| IBIS file imx8qx_17x17_v104.ibs generated by Viper version: 2017.04.12
[IBIS Ver]   6.0
[Comment Char] |_char
[File name]   imx8qxp_17x17_v104.ibs
[File Rev]   1.04
[Date]   Oct 18,2021
[Source]   NXP Viper 2017.04.12
[Notes]
[Disclaimer] IMPORTANT NOTICE
  This information is provided on an AS IS basis and without warranty.
  IN NO EVENT SHALL NXP BE LIABLE FOR INCIDENTAL OR CONSEQUENTIAL
  DAMAGES ARISING FROM USE OF THIS INFORMATION. THIS DISCLAIMER OF
  WARRANTY EXTENDS TO THE USER OF THE INFORMATION, AND TO THEIR CUSTOMERS
  OR USERS OF PRODUCTS  AND IS IN LIEU OF ALL WARRANTIES WHETHER EXPRESS,
  IMPLIED, OR STATUTORY, INCLUDING IMPLIED WARRANTIES OF MERCHANTABILITY
  OR FITNESS FOR PARTICULAR PURPOSE.
  NXP does not represent or warrant that the information furnished
  hereunder is free of infringement of any third party patents,
  copyrights, trade secrets, or other intellectual property rights.
  NXP does not represent or warrant that the information is free of
  defect, or that it meets any particular standard, requirements or need
  of the user of the infomation or their customers.
  NXP reserves the right to change the information in this file
  without notice.
   http://www.nxp.com
[Copyright]   (C) Copyright NXP 2006 - 2018, All Rights Reserved.
|   imx8qxp_17x17
[Component] imx8qxp_17x17_v104
[Manufacturer] NXP
[Package]
|   typ   min   max
R_pkg   0.31846   0.033582   0.75433
L_pkg   2.117e-9   3.409e-10   4.458e-9
C_pkg   1.134e-12   5.597e-13   3.274e-12
[Pin]   Signal_name   model_name   R_pin   L_pin   C_pin
A3   VSS_MAIN   GND   NA   NA   NA
A5   DDR_DCF18   PCKE_PAD   0.60598   3.663e-9   1.638e-12
A7   DDR_CK1_P   PCK_PAD   0.56666   3.47e-9   1.588e-12
A9   DDR_DCF26   PCKE_PAD   0.48689   3.01e-9   1.443e-12
A11   PCIE_CTRL0_PERST_B   3V3SF_1V8_3V3_FCGPIO   0.3033   2.06e-9   1.123e-12
A13   PCIE0_TX0_P   ABI_SERDES   0.34015   2.505e-9   1.009e-12
A15   PCIE0_RX0_P   ABI_SERDES   0.46929   3.272e-9   1.374e-12
A17   USB_OTG1_ID   USB_NXP   0.33178   2.305e-9   1.189e-12
A19   USB_OTG1_DP   USB_NXP   0.36817   2.72e-9   1.1e-12
A21   EMMC0_DATA0   3V3SF_1V8_3V3_FCGPIO   0.40744   2.664e-9   1.313e-12
A23   ENET0_RGMII_RXC   RGMIIRX_GPIO   0.31942   2.189e-9   1.146e-12
A25   ENET0_MDC   3V3SF_1V8_3V3_FCGPIO   0.32796   2.158e-9   1.166e-12
A27   VSS_MAIN   GND   NA   NA   NA
B2   DDR_DCF01   PCKE_PAD   0.68397   4.007e-9   1.734e-12
B4   DDR_DCF07   PCKE_PAD   0.58694   3.527e-9   1.632e-12
B6   DDR_DCF17   PCKE_PAD   0.52931   3.211e-9   1.459e-12
B8   DDR_CK1_N   PCK_PAD   0.59395   3.579e-9   1.611e-12
B10   DDR_DCF21   PCKE_PAD   0.75433   4.458e-9   1.957e-12
B12   PCIE0_TX0_N   ABI_SERDES   0.32805   2.401e-9   1.044e-12
B14   PCIE_CTRL0_WAKE_B   3V3SF_1V8_3V3_FCGPIO   0.37118   2.405e-9   1.258e-12
B16   PCIE0_RX0_N   ABI_SERDES   0.45484   3.105e-9   1.38e-12
B18   USB_OTG1_DN   USB_NXP   0.36895   2.655e-9   1.113e-12
B20   EMMC0_RESET_B   3V3SF_1V8_3V3_FCGPIO   0.3187   2.151e-9   1.117e-12
B22   ENET0_RGMII_TXD3   RGMIITX_GPIO   0.30644   2.133e-9   1.094e-12
B24   ENET0_RGMII_RXD3   RGMIIRX_GPIO   0.30222   2.062e-9   1.102e-12
B26   ESAI0_FSR   RGMIITX_GPIO   0.37989   2.442e-9   1.258e-12
B28   ESAI0_TX4_RX1   RGMIITX_GPIO   0.45602   2.794e-9   1.358e-12
C1   VSS_MAIN   GND   NA   NA   NA
C3   VSS_MAIN   GND   NA   NA   NA
C5   VSS_MAIN   GND   NA   NA   NA
C7   VSS_MAIN   GND   NA   NA   NA
C9   VSS_MAIN   GND   NA   NA   NA
C11   VSS_MAIN   GND   NA   NA   NA
C13   PCIE_REFCLK100M_N   PCIEREFCLKIO_N   0.32064   2.101e-9   1.131e-12
C15   VSS_MAIN   GND   NA   NA   NA
C17   VSS_MAIN   GND   NA   NA   NA
C19   VDD_EMMC0_VSELECT_1P8_3P3   POWER
C21   ENET0_RGMII_TXD1   RGMIITX_GPIO   0.25476   1.777e-9   1.026e-12
C23   ENET0_RGMII_RXD0   RGMIIRX_GPIO   0.28143   1.95e-9   1.063e-12
C25   ESAI0_SCKT   RGMIITX_GPIO   0.32741   2.164e-9   1.13e-12
C27   ESAI0_TX2_RX3   RGMIIRX_GPIO   0.48998   3.038e-9   1.422e-12
C29   VSS_MAIN   GND   NA   NA   NA
D2   DDR_DCF12   PCKE_PAD   0.71074   4.168e-9   1.828e-12
D4   DDR_DCF05   PCKE_PAD   0.5124   3.09e-9   1.489e-12
D6   DDR_DCF20   PCKE_PAD   0.53119   3.213e-9   1.505e-12
D8   DDR_DCF29   PCKE_PAD   0.35048   2.267e-9   1.192e-12
D10   DDR_DCF28   PCKE_PAD   0.4342   2.666e-9   1.32e-12
D12   VDD_USB_3P3   POWER
D14   PCIE_REFCLK100M_P   PCIEREFCLKIO_P   0.32297   2.08e-9   1.168e-12
D16   VDD_USB_SS3_LDO_1P0_CAP   POWER
D18   VDD_EMMC0_1P8_3P3   POWER
D20   VDD_ENET0_VSELECT_1P8_2P5_3P3   POWER
D22   ENET0_RGMII_RXD1   RGMIIRX_GPIO   0.1839   1.421e-9   8.563e-13
D24   ESAI0_TX3_RX2   RGMIIRX_GPIO   0.3864   2.495e-9   1.223e-12
D26   SPI3_CS0   3V3SF_1V8_3V3_FCGPIO   0.54046   3.334e-9   1.559e-12
D28   SPI3_SCK   3V3SF_1V8_3V3_FCGPIO   0.38925   2.486e-9   1.254e-12
E1   DDR_DCF15   PCKE_PAD   0.65321   3.867e-9   1.722e-12
E3   DDR_DCF03   PCKE_PAD   0.50795   3.087e-9   1.474e-12
E5   DDR_DCF22   PCKE_PAD   0.48237   2.951e-9   1.392e-12
E7   DDR_DCF32   PCKE_PAD   0.33907   2.197e-9   1.192e-12
E9   DDR_DCF27   PCKE_PAD   0.32561   2.108e-9   1.154e-12
E11   PCIE_CTRL0_CLKREQ_B   3V3SF_1V8_3V3_FCGPIO   0.16383   1.294e-9   8.23e-13
E13   EMMC0_CMD   3V3SF_1V8_3V3_FCGPIO   0.1937   1.633e-9   9.088e-13
E15   EMMC0_DATA6   3V3SF_1V8_3V3_FCGPIO   0.3561   2.314e-9   1.223e-12
E17   VSS_MAIN   GND   NA   NA   NA
E19   EMMC0_DATA3   3V3SF_1V8_3V3_FCGPIO   0.2151   1.54e-9   8.782e-13
E21   VDD_ENET0_1P8_2P5_3P3   POWER
E23   ESAI0_FST   RGMIITX_GPIO   0.19585   1.448e-9   9.33e-13
E25   ESAI0_TX1   RGMIIRX_GPIO   0.29822   1.981e-9   1.079e-12
E27   SPDIF0_EXT_CLK   RGMIITX_GPIO   0.34327   2.258e-9   1.153e-12
E29   UART1_RX   3V3SF_1V8_3V3_FCGPIO   0.43258   2.758e-9   1.353e-12
F2   VSS_MAIN   GND   NA   NA   NA
F4   VSS_MAIN   GND   NA   NA   NA
F6   VSS_MAIN   GND   NA   NA   NA
F8   VSS_MAIN   GND   NA   NA   NA
F10   DDR_ZQ   NC   0.20708   1.713e-9   1.28e-12
F12   PCIE_REF_QR   NC   0.17551   1.316e-9   9.358e-13
F14   EMMC0_CLK   3V3SF_1V8_3V3_FCGPIO   0.1708   1.429e-9   8.15e-13
F16   EMMC0_DATA5   3V3SF_1V8_3V3_FCGPIO   0.12694   1.075e-9   7.546e-13
F18   EMMC0_DATA1   3V3SF_1V8_3V3_FCGPIO   0.16418   1.28e-9   8.764e-13
F20   ENET0_RGMII_TXD0   RGMIITX_GPIO   0.19161   1.414e-9   8.951e-13
F22   ENET0_REFCLK_125M_25M   3V3SF_1V8_3V3_FCGPIO   0.16413   1.301e-9   7.971e-13
F24   SPDIF0_RX   RGMIIRX_GPIO   0.28282   1.891e-9   1.046e-12
F26   VDD_ENET_MDIO_1P8_3P3   POWER
F28   SPI3_CS1   3V3SF_1V8_3V3_FCGPIO   0.35831   2.326e-9   1.185e-12
G1   DDR_DCF10   PCKE_PAD   0.65109   3.855e-9   1.688e-12
G3   DDR_CK0_N   PCK_PAD   0.55273   3.295e-9   1.525e-12
G5   DDR_DCF00   PCKE_PAD   0.49032   2.993e-9   1.45e-12
G7   DDR_DCF33   PCKE_PAD   0.31582   2.024e-9   1.17e-12
G9   DDR_DCF31   PCKE_PAD   0.3963   2.501e-9   1.183e-12
G11   PCIE0_PHY_PLL_REF_RETURN   GND   0.033582   5.677e-10   1.252e-12
G13   USB_SS3_TC1   3V3SF_3V3_FCGPIO   0.11957   1.018e-9   7.88e-13
G15   EMMC0_DATA2   3V3SF_1V8_3V3_FCGPIO   0.14436   1.152e-9   7.231e-13
G17   EMMC0_DATA4   3V3SF_1V8_3V3_FCGPIO   0.14044   1.144e-9   8.112e-13
G19   ENET0_RGMII_TXC   RGMIITX_GPIO   0.14473   1.165e-9   8.155e-13
G21   ENET0_RGMII_RXD2   RGMIIRX_GPIO   0.14641   1.239e-9   7.478e-13
G23   ESAI0_TX0   RGMIIRX_GPIO   0.21582   1.512e-9   9.211e-13
G25   SPI3_SDO   3V3SF_1V8_3V3_FCGPIO   0.28321   1.89e-9   1.032e-12
G27   UART1_CTS_B   3V3SF_1V8_3V3_FCGPIO   0.34681   2.245e-9   1.16e-12
G29   UART1_RTS_B   3V3SF_1V8_3V3_FCGPIO   0.37578   2.468e-9   1.258e-12
H2   DDR_CK0_P   PCK_PAD   0.51499   3.138e-9   1.476e-12
H4   DDR_DCF24   PCKE_PAD   0.37984   2.355e-9   1.21e-12
H6   DDR_DCF19   PCKE_PAD   0.34619   2.213e-9   1.204e-12
H8   DDR_DCF30   PCKE_PAD   0.24305   1.688e-9   1.007e-12
H10   DDR_DCF25   PCKE_PAD   0.32921   2.167e-9   1.178e-12
H12   PCIE_REXT   NC   0.093831   8.543e-10   6.92e-13
H14   USB_SS3_TC3   3V3SF_3V3_FCGPIO   0.11822   1.017e-9   7.579e-13
H16   EMMC0_DATA7   3V3SF_1V8_3V3_FCGPIO   0.08452   8.213e-10   7.472e-13
H18   ENET0_RGMII_TX_CTL   RGMIITX_GPIO   0.046311   6.292e-10   5.597e-13
H20   ENET0_RGMII_RX_CTL   RGMIIRX_GPIO   0.19545   1.425e-9   8.908e-13
H22   ESAI0_SCKR   RGMIITX_GPIO   0.16182   1.249e-9   7.9e-13
H24   SPI3_SDI   3V3SF_1V8_3V3_FCGPIO   0.29834   1.966e-9   1.068e-12
H26   VSS_MAIN   GND   NA   NA   NA
H28   SPI0_CS0   3V3SF_1V8_3V3_FCGPIO   0.42978   2.766e-9   1.304e-12
J1   VSS_MAIN   GND   NA   NA   NA
J3   VSS_MAIN   GND   NA   NA   NA
J5   VSS_MAIN   GND   NA   NA   NA
J7   VSS_MAIN   GND   NA   NA   NA
J9   VDD_PCIE_DIG_1P8_3P3   POWER
J11   VDD_PCIE_1P8   POWER
J13   VSS_MAIN   GND   NA   NA   NA
J15   USB_OTG1_VBUS   USB_NXP   0.13315   1.223e-9   6.609e-13
J17   EMMC0_STROBE   3V3SF_1V8_3V3_FCGPIO   0.074471   7.722e-10   6.943e-13
J19   ENET0_RGMII_TXD2   RGMIITX_GPIO   0.038799   3.409e-10   6.494e-13
J21   ENET0_MDIO   3V3SF_1V8_3V3_FCGPIO   0.10797   9.439e-10   7.106e-13
J23   SPDIF0_TX   RGMIIRX_GPIO   0.22123   1.614e-9   9.35e-13
J25   UART1_TX   3V3SF_1V8_3V3_FCGPIO   0.30141   1.998e-9   1.09e-12
J27   SPI0_SDO   3V3SF_1V8_3V3_FCGPIO   0.31847   2.065e-9   1.139e-12
J29   SPI0_SDI   3V3SF_1V8_3V3_FCGPIO   0.34645   2.267e-9   1.203e-12
K2   DDR_DCF08   PCKE_PAD   0.47957   2.948e-9   1.473e-12
K4   DDR_DCF14   PCKE_PAD   0.4787   2.939e-9   1.452e-12
K6   DDR_DCF04   PCKE_PAD   0.25956   1.689e-9   9.947e-13
K8   VDD_DDR_VDDQ   POWER
K10   VDD_ANA0_1P8   POWER
K12   VDD_PCIE_LDO_1P0_CAP   POWER
K14   VDD_USB_1P8   POWER
K16   VDD_MAIN   POWER
K18   VSS_MAIN   GND   NA   NA   NA
K20   VDD_GPU   POWER
K22   ESAI0_TX5_RX0   RGMIITX_GPIO   0.18734   1.405e-9   8.834e-13
K24   MCLK_OUT0   3V3SF_1V8_3V3_FCGPIO   0.27272   1.839e-9   1.066e-12
K26   VDD_ESAI_SPDIF_1P8_2P5_3P3   POWER
K28   SPI0_CS1   3V3SF_1V8_3V3_FCGPIO   0.32295   2.115e-9   1.146e-12
L1   DDR_DCF11   PCKE_PAD   0.39285   2.474e-9   1.275e-12
L3   DDR_DCF09   PCKE_PAD   0.43975   2.731e-9   1.384e-12
L5   DDR_DCF23   PCKE_PAD   0.25824   1.745e-9   1.009e-12
L7   DDR_DCF16   PCKE_PAD   0.25409   1.709e-9   9.506e-13
L9   VSS_MAIN   GND   NA   NA   NA
L11   VSS_MAIN   GND   NA   NA   NA
L13   VDD_MAIN   POWER
L15   VSS_MAIN   GND   NA   NA   NA
L17   VDD_GPU   POWER
L19   VDD_GPU   POWER
L21   VDD_MAIN   POWER
L23   MCLK_IN0   3V3SF_1V8_3V3_FCGPIO   0.14369   1.143e-9   7.893e-13
L25   SPI0_SCK   3V3SF_1V8_3V3_FCGPIO   0.19113   1.427e-9   9.442e-13
L27   VDD_SPI_MCLK_UART_1P8_3P3   POWER
L29   VSS_MAIN   GND   NA   NA   NA
M2   VSS_MAIN   GND   NA   NA   NA
M4   VSS_MAIN   GND   NA   NA   NA
M6   VSS_MAIN   GND   NA   NA   NA
M8   VDD_DDR_VDDQ   POWER
M10   VDD_MAIN   POWER
M12   VSS_MAIN   GND   NA   NA   NA
M14   VDD_MAIN   POWER
M16   VSS_MAIN   GND   NA   NA   NA
M18   VDD_GPU   POWER
M20   VSS_MAIN   GND   NA   NA   NA
M22   MCLK_IN1   3V3SF_1V8_3V3_FCGPIO   0.10409   9.11e-10   7.793e-13
M24   VSS_MAIN   GND   NA   NA   NA
M26   VSS_MAIN   GND   NA   NA   NA
M28   ADC_VREFH   POWER   0.19187   1.497e-9   1.547e-12
N1   DDR_DQ02   PDDRIO_PAD   0.55563   3.352e-9   1.521e-12
N3   DDR_DQ00   PDDRIO_PAD   0.50424   3.21e-9   1.442e-12
N5   DDR_DQ13   PDDRIO_PAD   0.45478   2.757e-9   1.37e-12
N7   DDR_DQ15   PDDRIO_PAD   0.35806   2.282e-9   1.073e-12
N9   VDD_DDR_VDDQ   POWER
N11   VDD_MAIN   POWER
N13   VSS_MAIN   GND   NA   NA   NA
N15   VDD_MAIN   POWER
N17   VSS_MAIN   GND   NA   NA   NA
N19   VDD_GPU   POWER
N21   VSS_MAIN   GND   NA   NA   NA
N23   ADC_IN1   CSF_1V8_FCGPIO   0.15303   1.165e-9   8.275e-13
N25   ADC_IN3   CSF_1V8_FCGPIO   0.26276   1.717e-9   9.703e-13
N27   ADC_IN2   CSF_1V8_FCGPIO   0.25756   1.755e-9   9.937e-13
N29   ADC_VREFL   GND   0.17561   1.455e-9   1.639e-12
P2   DDR_DQ01   PDDRIO_PAD   0.40818   2.601e-9   1.24e-12
P4   DDR_DQ12   PDDRIO_PAD   0.31857   2.054e-9   1.081e-12
P6   DDR_DQ14   PDDRIO_PAD   0.32363   2.082e-9   1.079e-12
P8   VDD_DDR_VDDQ   POWER
P10   VSS_MAIN   GND   NA   NA   NA
P12   VDD_MAIN   POWER
P14   VSS_MAIN   GND   NA   NA   NA
P16   VDD_MAIN   POWER
P18   VSS_MAIN   GND   NA   NA   NA
P20   VDD_GPU   POWER
P22   VDD_ADC_1P8   POWER
P24   ADC_IN0   CSF_1V8_FCGPIO   0.17153   1.276e-9   8.767e-13
P26   ADC_IN5   CSF_1V8_FCGPIO   0.23782   1.642e-9   9.683e-13
P28   ADC_IN4   CSF_1V8_FCGPIO   0.27134   1.832e-9   1.061e-12
R1   VSS_MAIN   GND   NA   NA   NA
R3   VSS_MAIN   GND   NA   NA   NA
R5   VSS_MAIN   GND   NA   NA   NA
R7   VSS_MAIN   GND   NA   NA   NA
R9   VSS_MAIN   GND   NA   NA   NA
R11   VSS_MAIN   GND   NA   NA   NA
R13   VDD_MAIN   POWER
R15   VSS_MAIN   GND   NA   NA   NA
R17   VDD_GPU   POWER
R19   VSS_MAIN   GND   NA   NA   NA
R21   VDD_MAIN   POWER
R23   VSS_MAIN   GND   NA   NA   NA
R25   VSS_MAIN   GND   NA   NA   NA
R27   VSS_MAIN   GND   NA   NA   NA
R29   VSS_MAIN   GND   NA   NA   NA
T2   DDR_DQ03   PDDRIO_PAD   0.37672   2.394e-9   1.21e-12
T4   DDR_DQS1_N   PDQS_PAD   0.33781   2.201e-9   1.025e-12
T6   DDR_DM1   PDDRIO_PAD   0.16039   1.193e-9   7.698e-13
T8   VDD_DDR_VDDQ   POWER
T10   VDD_MAIN   POWER
T12   VSS_MAIN   GND   NA   NA   NA
T14   VDD_MAIN   POWER
T16   VSS_MAIN   GND   NA   NA   NA
T18   VDD_GPU   POWER
T20   VSS_MAIN   GND   NA   NA   NA
T22   FLEXCAN0_RX   3V3SF_1V8_3V3_FCGPIO   0.35436   2.283e-9   1.246e-12
T24   FLEXCAN1_RX   3V3SF_1V8_3V3_FCGPIO   0.27694   1.832e-9   1.042e-12
T26   VDD_ADC_DIG_1P8   POWER
T28   FLEXCAN2_RX   3V3SF_1V8_3V3_FCGPIO   0.2951   1.929e-9   1.093e-12
U1   DDR_DQS0_N   PDQS_PAD   0.50661   3.092e-9   1.537e-12
U3   DDR_DQS0_P   PDQS_PAD   0.53219   3.191e-9   1.464e-12
U5   DDR_DQS1_P   PDQS_PAD   0.31801   2.083e-9   1.001e-12
U7   DDR_DTO0   PDDRIO_PAD   0.098895   8.797e-10   7.121e-13
U9   VDD_DDR_VDDQ   POWER
U11   VDD_MAIN   POWER
U13   VSS_MAIN   GND   NA   NA   NA
U15   VDD_MAIN   POWER
U17   VSS_MAIN   GND   NA   NA   NA
U19   VDD_MAIN   POWER
U21   VDD_CAN_UART_1P8_3P3   POWER
U23   UART0_TX   3V3SF_1V8_3V3_FCGPIO   0.19876   1.443e-9   8.795e-13
U25   FLEXCAN0_TX   3V3SF_1V8_3V3_FCGPIO   0.31323   2.004e-9   1.087e-12
U27   FLEXCAN2_TX   3V3SF_1V8_3V3_FCGPIO   0.24294   1.671e-9   8.827e-13
U29   FLEXCAN1_TX   3V3SF_1V8_3V3_FCGPIO   0.27629   1.907e-9   1.1e-12
V2   VSS_MAIN   GND   NA   NA   NA
V4   VSS_MAIN   GND   NA   NA   NA
V6   VSS_MAIN   GND   NA   NA   NA
V8   VDD_DDR_VDDQ   POWER
V10   VSS_MAIN   GND   NA   NA   NA
V12   VDD_A35   POWER
V14   VDD_A35   POWER
V16   VDD_A35   POWER
V18   VSS_MAIN   GND   NA   NA   NA
V20   VDD_MAIN   POWER
V22   MIPI_DSI0_I2C0_SDA   3V3SF_1V8_3V3_FCGPIO   0.076086   7.914e-10   6.572e-13
V24   VSS_MAIN   GND   NA   NA   NA
V26   UART2_TX   3V3SF_1V8_3V3_FCGPIO   0.17121   1.271e-9   8.781e-13
V28   UART0_RX   3V3SF_1V8_3V3_FCGPIO   0.26081   1.794e-9   9.544e-13
W1   DDR_DM0   PDDRIO_PAD   0.35899   2.276e-9   1.198e-12
W3   DDR_DQ10   PDDRIO_PAD   0.23291   1.571e-9   8.963e-13
W5   DDR_ATO   NC   0.37202   2.325e-9   1.123e-12
W7   VDD_DDR_PLL_1P8   POWER
W9   VSS_MAIN   GND   NA   NA   NA
W11   VSS_MAIN   GND   NA   NA   NA
W13   VDD_A35   POWER
W15   VDD_A35   POWER
W17   VDD_A35   POWER
W19   VSS_MAIN   GND   NA   NA   NA
W21   VDD_ANA1_1P8   POWER
W23   JTAG_TMS   CSF_1V8_FCGPIO   0.17649   1.322e-9   8.415e-13
W25   MIPI_DSI1_I2C0_SDA   3V3SF_1V8_3V3_FCGPIO   0.18746   1.357e-9   8.589e-13
W27   MIPI_DSI0_I2C0_SCL   3V3SF_1V8_3V3_FCGPIO   0.21768   1.557e-9   9.53e-13
W29   UART2_RX   3V3SF_1V8_3V3_FCGPIO   0.30148   2.093e-9   1.126e-12
Y2   DDR_DQ04   PDDRIO_PAD   0.33834   2.165e-9   1.187e-12
Y4   DDR_DQ08   PDDRIO_PAD   0.18397   1.396e-9   8.449e-13
Y6   DDR_VREF   POWER   0.047878   4.824e-10   3.274e-12
Y8   VDD_DDR_VDDQ   POWER
Y10   VDD_MAIN   POWER
Y12   VSS_MAIN   GND   NA   NA   NA
Y14   VDD_MAIN   POWER
Y16   VSS_MAIN   GND   NA   NA   NA
Y18   VDD_MAIN   POWER
Y20   VSS_MAIN   GND   NA   NA   NA
Y22   SCU_GPIO0_00   CSF_1V8_FCGPIO   0.14821   1.137e-9   8.116e-13
Y24   JTAG_TDO   CSF_1V8_FCGPIO   0.27697   1.856e-9   1.043e-12
Y26   VDD_SNVS_4P2   POWER
Y28   MIPI_DSI1_I2C0_SCL   3V3SF_1V8_3V3_FCGPIO   0.27823   1.915e-9   1.042e-12
AA1   VSS_MAIN   GND   NA   NA   NA
AA3   VSS_MAIN   GND   NA   NA   NA
AA5   VSS_MAIN   GND   NA   NA   NA
AA7   VSS_MAIN   GND   NA   NA   NA
AA9   VDD_DDR_VDDQ   POWER
AA11   VDD_MAIN   POWER
AA13   VDD_MIPI_1P8   POWER
AA15   VDD_MIPI_1P0   POWER
AA17   VSS_MAIN   GND   NA   NA   NA
AA19   VDD_MAIN   POWER
AA21   VDD_TMPR_CSI_1P8_3P3   POWER
AA23   PMIC_INT_B   CSF_1V8_FCGPIO   0.23793   1.675e-9   9.771e-13
AA25   TEST_MODE_SELECT   CSF_1V8_FCGPIO   0.25321   1.727e-9   9.528e-13
AA27   VSS_MAIN   GND   NA   NA   NA
AA29   JTAG_TCK   CSF_1V8_FCGPIO   0.32393   2.149e-9   1.169e-12
AB2   DDR_DQ05   PDDRIO_PAD   0.31478   1.975e-9   1.073e-12
AB4   DDR_DQ11   PDDRIO_PAD   0.31536   2.062e-9   1.079e-12
AB6   DDR_DTO1   PDDRIO_PAD   0.30358   1.978e-9   1.084e-12
AB8   VDD_DDR_VDDQ   POWER
AB10   QSPI0A_DQS   3V3SF_1V8_3V3_FCGPIO   0.16544   1.252e-9   7.974e-13
AB12   QSPI0A_SS0_B   3V3SF_1V8_3V3_FCGPIO   0.12301   1.068e-9   7.379e-13
AB14   VDD_MIPI_1P8   POWER
AB16   VDD_MIPI_1P0   POWER
AB18   VDD_MIPI_CSI_DIG_1P8   POWER
AB20   PMIC_ON_REQ   IO_20UM_RES_ANAF_1V8   0.25377   1.732e-9   1.015e-12
AB22   SCU_BOOT_MODE3   CSF_1V8_FCGPIO   0.14142   1.539e-9   7.172e-13
AB24   SCU_PMIC_STANDBY   CSF_1V8_FCGPIO   0.39697   2.526e-9   1.282e-12
AB26   VDD_SNVS_LDO_1P8_CAP   POWER
AB28   JTAG_TRST_B   CSF_1V8_FCGPIO   0.2837   1.928e-9   1.052e-12
AC1   DDR_DQ06   PDDRIO_PAD   0.34319   2.15e-9   1.174e-12
AC3   DDR_DQ07   PDDRIO_PAD   0.30034   1.943e-9   9.997e-13
AC5   DDR_DQ09   PDDRIO_PAD   0.27828   1.992e-9   9.843e-13
AC7   QSPI0B_DATA0   3V3SF_1V8_3V3_FCGPIO   0.20931   1.491e-9   9.385e-13
AC9   QSPI0A_DATA2   3V3SF_1V8_3V3_FCGPIO   0.19074   1.515e-9   8.42e-13
AC11   MIPI_CSI0_DATA3_N   MIPI_CSI   0.36497   2.357e-9   1.219e-12
AC13   MIPI_CSI0_DATA1_N   MIPI_CSI   0.37028   2.387e-9   1.176e-12
AC15   MIPI_CSI0_CLK_N   MIPI_CSI   0.33094   2.141e-9   1.162e-12
AC17   MIPI_CSI0_DATA0_N   MIPI_CSI   0.3426   2.262e-9   1.078e-12
AC19   MIPI_CSI0_DATA2_N   MIPI_CSI   0.34464   2.341e-9   1.202e-12
AC21   CSI_D00   IO_20UM_RES_ANAF   0.2875   1.926e-9   1.045e-12
AC23   SCU_BOOT_MODE1   CSF_1V8_FCGPIO   0.46828   3.067e-9   1.28e-12
AC25   SCU_GPIO0_01   CSF_1V8_FCGPIO   0.28162   1.859e-9   9.376e-13
AC27   PMIC_I2C_SCL   CSF_1V8_FCGPIO   0.29178   1.969e-9   9.85e-13
AC29   JTAG_TDI   CSF_1V8_FCGPIO   0.36581   2.383e-9   1.201e-12
AD2   VSS_MAIN   GND   NA   NA   NA
AD4   VSS_MAIN   GND   NA   NA   NA
AD6   VSS_MAIN   GND   NA   NA   NA
AD8   VDD_QSPI0A_1P8_3P3   POWER
AD10   QSPI0A_SS1_B   3V3SF_1V8_3V3_FCGPIO   0.21596   1.516e-9   9.282e-13
AD12   MIPI_CSI0_DATA3_P   MIPI_CSI   0.36604   2.336e-9   1.269e-12
AD14   MIPI_CSI0_DATA1_P   MIPI_CSI   0.35133   2.266e-9   1.16e-12
AD16   MIPI_CSI0_CLK_P   MIPI_CSI   0.31792   2.092e-9   1.089e-12
AD18   MIPI_CSI0_DATA0_P   MIPI_CSI   0.33148   2.205e-9   1.186e-12
AD20   MIPI_CSI0_DATA2_P   MIPI_CSI   0.35486   2.319e-9   1.155e-12
AD22   CSI_D02   IO_20UM_RES_ANAF   0.18011   1.338e-9   8.479e-13
AD24   VSS_MAIN   GND   NA   NA   NA
AD26   SCU_BOOT_MODE0   CSF_1V8_FCGPIO   0.26532   1.766e-9   1.036e-12
AD28   POR_B   CSF_1V8_FCGPIO   0.33136   2.163e-9   1.143e-12
AE1   QSPI0B_DATA1   3V3SF_1V8_3V3_FCGPIO   0.43816   2.72e-9   1.339e-12
AE3   QSPI0B_DATA3   3V3SF_1V8_3V3_FCGPIO   0.34172   2.199e-9   1.163e-12
AE5   VDD_QSPI0B_1P8_3P3   POWER
AE7   QSPI0B_SS0_B   3V3SF_1V8_3V3_FCGPIO   0.24295   1.662e-9   9.832e-13
AE9   VSS_MAIN   GND   NA   NA   NA
AE11   VSS_MAIN   GND   NA   NA   NA
AE13   VSS_MAIN   GND   NA   NA   NA
AE15   VSS_MAIN   GND   NA   NA   NA
AE17   VSS_MAIN   GND   NA   NA   NA
AE19   VSS_MAIN   GND   NA   NA   NA
AE21   VSS_MAIN   GND   NA   NA   NA
AE23   ANA_TEST_OUT_P   NC   0.24109   1.768e-9   8.791e-13
AE25   SCU_BOOT_MODE2   CSF_1V8_FCGPIO   0.41153   2.694e-9   1.288e-12
AE27   VSS_MAIN   GND   NA   NA   NA
AE29   PMIC_I2C_SDA   CSF_1V8_FCGPIO   0.42834   2.703e-9   1.339e-12
AF2   QSPI0B_DATA2   3V3SF_1V8_3V3_FCGPIO   0.37719   2.419e-9   1.237e-12
AF4   QSPI0B_DQS   3V3SF_1V8_3V3_FCGPIO   0.30699   2.036e-9   1.154e-12
AF6   QSPI0B_SS1_B   3V3SF_1V8_3V3_FCGPIO   0.36204   2.294e-9   1.201e-12
AF8   MIPI_DSI1_DATA0_N   MIPI_LVDS_DSI   0.37839   2.428e-9   1.277e-12
AF10   MIPI_DSI1_DATA1_N   MIPI_LVDS_DSI   0.36272   2.34e-9   1.211e-12
AF12   MIPI_DSI0_DATA3_N   MIPI_LVDS_DSI   0.3616   2.356e-9   1.209e-12
AF14   MIPI_DSI0_CLK_N   MIPI_LVDS_DSI   0.3301   2.168e-9   1.148e-12
AF16   MIPI_DSI0_DATA2_N   MIPI_LVDS_DSI   0.33145   2.163e-9   1.152e-12
AF18   MIPI_CSI0_MCLK_OUT   CSF_1V8_FCGPIO   0.30216   1.966e-9   1.115e-12
AF20   CSI_VSYNC   IO_20UM_RES_ANAF   0.25355   1.811e-9   9.414e-13
AF22   VDD_CSI_1P8_3P3   POWER
AF24   ANA_TEST_OUT_N   NC   0.25249   1.72e-9   9.774e-13
AF26   RTC_XTALO   IO_20UM_RES_ANAF_1V8   0.2789   1.885e-9   1.06e-12
AF28   XTALO   IO_20UM_RES_ANAF_1V8   0.39297   2.475e-9   1.274e-12
AG1   VSS_MAIN   GND   NA   NA   NA
AG3   QSPI0A_SCLK   3V3SF_1V8_3V3_FCGPIO   0.48374   2.971e-9   1.409e-12
AG5   QSPI0A_DATA3   3V3SF_1V8_3V3_FCGPIO   0.35396   2.317e-9   1.193e-12
AG7   MIPI_DSI1_DATA2_N   MIPI_LVDS_DSI   0.42191   2.679e-9   1.329e-12
AG9   MIPI_DSI1_CLK_N   MIPI_LVDS_DSI   0.39245   2.544e-9   1.298e-12
AG11   MIPI_DSI1_DATA3_N   MIPI_LVDS_DSI   0.36671   2.41e-9   1.194e-12
AG13   MIPI_DSI0_DATA1_N   MIPI_LVDS_DSI   0.34731   2.34e-9   1.17e-12
AG15   MIPI_DSI0_DATA0_N   MIPI_LVDS_DSI   0.33429   2.207e-9   1.146e-12
AG17   VSS_MAIN   GND   NA   NA   NA
AG19   CSI_PCLK   3V3SF_1V8_3V3_FCGPIO   0.28612   2.024e-9   1.02e-12
AG21   CSI_D04   IO_20UM_RES_ANAF   0.24994   1.78e-9   1.018e-12
AG23   CSI_D03   IO_20UM_RES_ANAF   0.25608   1.84e-9   9.907e-13
AG25   VSS_MAIN   GND   NA   NA   NA
AG27   VSS_MAIN   GND   NA   NA   NA
AG29   VSS_MAIN   GND   NA   NA   NA
AH2   QSPI0B_SCLK   3V3SF_1V8_3V3_FCGPIO   0.48208   2.96e-9   1.432e-12
AH4   QSPI0A_DATA1   3V3SF_1V8_3V3_FCGPIO   0.44092   2.815e-9   1.339e-12
AH6   VSS_MAIN   GND   NA   NA   NA
AH8   MIPI_DSI1_DATA0_P   MIPI_LVDS_DSI   0.38646   2.565e-9   1.234e-12
AH10   MIPI_DSI1_DATA1_P   MIPI_LVDS_DSI   0.3636   2.493e-9   1.219e-12
AH12   MIPI_DSI0_DATA3_P   MIPI_LVDS_DSI   0.35841   2.451e-9   1.16e-12
AH14   MIPI_DSI0_CLK_P   MIPI_LVDS_DSI   0.32989   2.222e-9   1.147e-12
AH16   MIPI_DSI0_DATA2_P   MIPI_LVDS_DSI   0.33366   2.227e-9   1.158e-12
AH18   CSI_RESET   3V3SF_1V8_3V3_FCGPIO   0.32447   2.187e-9   1.155e-12
AH20   CSI_HSYNC   IO_20UM_RES_ANAF   0.27429   1.939e-9   1.036e-12
AH22   CSI_D07   IO_20UM_RES_ANAF   0.28957   2.007e-9   1.077e-12
AH24   CSI_D01   IO_20UM_RES_ANAF   0.31604   2.206e-9   1.07e-12
AH26   RTC_XTALI   IO_20UM_RES_ANAF_1V8   0.34993   2.421e-9   1.131e-12
AH28   XTALI   IO_20UM_RES_ANAF_1V8   0.4205   2.629e-9   1.289e-12
AJ3   VSS_MAIN   GND   NA   NA   NA
AJ5   QSPI0A_DATA0   3V3SF_1V8_3V3_FCGPIO   0.41463   2.622e-9   1.323e-12
AJ7   MIPI_DSI1_DATA2_P   MIPI_LVDS_DSI   0.42097   2.693e-9   1.334e-12
AJ9   MIPI_DSI1_CLK_P   MIPI_LVDS_DSI   0.39887   2.692e-9   1.296e-12
AJ11   MIPI_DSI1_DATA3_P   MIPI_LVDS_DSI   0.36426   2.501e-9   1.239e-12
AJ13   MIPI_DSI0_DATA1_P   MIPI_LVDS_DSI   0.34325   2.375e-9   1.196e-12
AJ15   MIPI_DSI0_DATA0_P   MIPI_LVDS_DSI   0.32319   2.224e-9   1.165e-12
AJ17   CSI_EN   3V3SF_1V8_3V3_FCGPIO   0.40826   2.716e-9   1.29e-12
AJ19   CSI_MCLK   3V3SF_1V8_3V3_FCGPIO   0.33181   2.241e-9   1.197e-12
AJ21   CSI_D06   IO_20UM_RES_ANAF   0.30705   2.16e-9   1.092e-12
AJ23   CSI_D05   IO_20UM_RES_ANAF   0.35335   2.423e-9   1.173e-12
AJ25   ON_OFF_BUTTON   IO_20UM_RES_ANAF_1V8   0.37037   2.428e-9   1.197e-12
AJ27   VSS_MAIN   GND   NA   NA   NA
[Pin Mapping]   pulldown_ref   pullup_ref   gnd_clamp_ref   power_clamp_ref
A3   GND   NC   NC   NC
A5   GND   VDD_DDR_VDDQ   GND   VDD_DDR_VDDQ
A7   GND   VDD_DDR_VDDQ   GND   VDD_DDR_VDDQ
A9   GND   VDD_DDR_VDDQ   GND   VDD_DDR_VDDQ
A11   GND   VDD_PCIE_DIG_1P   GND   VDD_PCIE_DIG_1P
A13   GND   VDD_PCIE_LDO_1P   GND   VDD_PCIE_LDO_1P
A15   GND   VDD_PCIE_LDO_1P   GND   VDD_PCIE_LDO_1P
A17   GND   VDD_USB_1P8   GND   VDD_USB_1P8
A19   GND   VDD_USB_1P8   GND   VDD_USB_1P8
A21   GND   VDD_EMMC0_1P8_3   GND   VDD_EMMC0_1P8_3
A23   GND   VDD_ENET0_1P8_2   GND   VDD_ENET0_1P8_2
A25   GND   VDD_ENET_MDIO_1   GND   VDD_ENET_MDIO_1
A27   GND   NC   NC   NC
B2   GND   VDD_DDR_VDDQ   GND   VDD_DDR_VDDQ
B4   GND   VDD_DDR_VDDQ   GND   VDD_DDR_VDDQ
B6   GND   VDD_DDR_VDDQ   GND   VDD_DDR_VDDQ
B8   GND   VDD_DDR_VDDQ   GND   VDD_DDR_VDDQ
B10   GND   VDD_DDR_VDDQ   GND   VDD_DDR_VDDQ
B12   GND   VDD_PCIE_LDO_1P   GND   VDD_PCIE_LDO_1P
B14   GND   VDD_PCIE_DIG_1P   GND   VDD_PCIE_DIG_1P
B16   GND   VDD_PCIE_LDO_1P   GND   VDD_PCIE_LDO_1P
B18   GND   VDD_USB_1P8   GND   VDD_USB_1P8
B20   GND   VDD_EMMC0_VSELE   GND   VDD_EMMC0_VSELE
B22   GND   VDD_ENET0_VSELE   GND   VDD_ENET0_VSELE
B24   GND   VDD_ENET0_1P8_2   GND   VDD_ENET0_1P8_2
B26   GND   VDD_ESAI_SPDIF_   GND   VDD_ESAI_SPDIF_
B28   GND   VDD_ESAI_SPDIF_   GND   VDD_ESAI_SPDIF_
C1   GND   NC   NC   NC
C3   GND   NC   NC   NC
C5   GND   NC   NC   NC
C7   GND   NC   NC   NC
C9   GND   NC   NC   NC
C11   GND   NC   NC   NC
C13   GND   VDD_PCIE_1P8   GND   VDD_PCIE_1P8
C15   GND   NC   NC   NC
C17   GND   NC   NC   NC
C19   NC   VDD_EMMC0_VSELE   NC   NC
C21   GND   VDD_ENET0_VSELE   GND   VDD_ENET0_VSELE
C23   GND   VDD_ENET0_1P8_2   GND   VDD_ENET0_1P8_2
C25   GND   VDD_ESAI_SPDIF_   GND   VDD_ESAI_SPDIF_
C27   GND   VDD_ESAI_SPDIF_   GND   VDD_ESAI_SPDIF_
C29   GND   NC   NC   NC
D2   GND   VDD_DDR_VDDQ   GND   VDD_DDR_VDDQ
D4   GND   VDD_DDR_VDDQ   GND   VDD_DDR_VDDQ
D6   GND   VDD_DDR_VDDQ   GND   VDD_DDR_VDDQ
D8   GND   VDD_DDR_VDDQ   GND   VDD_DDR_VDDQ
D10   GND   VDD_DDR_VDDQ   GND   VDD_DDR_VDDQ
D12   NC   VDD_USB_3P3   NC   NC
D14   GND   VDD_PCIE_1P8   GND   VDD_PCIE_1P8
D16   NC   VDD_USB_SS3_LDO   NC   NC
D18   NC   VDD_EMMC0_1P8_3   NC   NC
D20   NC   VDD_ENET0_VSELE   NC   NC
D22   GND   VDD_ENET0_1P8_2   GND   VDD_ENET0_1P8_2
D24   GND   VDD_ESAI_SPDIF_   GND   VDD_ESAI_SPDIF_
D26   GND   VDD_SPI_MCLK_UA   GND   VDD_SPI_MCLK_UA
D28   GND   VDD_SPI_MCLK_UA   GND   VDD_SPI_MCLK_UA
E1   GND   VDD_DDR_VDDQ   GND   VDD_DDR_VDDQ
E3   GND   VDD_DDR_VDDQ   GND   VDD_DDR_VDDQ
E5   GND   VDD_DDR_VDDQ   GND   VDD_DDR_VDDQ
E7   GND   VDD_DDR_VDDQ   GND   VDD_DDR_VDDQ
E9   GND   VDD_DDR_VDDQ   GND   VDD_DDR_VDDQ
E11   GND   VDD_PCIE_DIG_1P   GND   VDD_PCIE_DIG_1P
E13   GND   VDD_EMMC0_1P8_3   GND   VDD_EMMC0_1P8_3
E15   GND   VDD_EMMC0_VSELE   GND   VDD_EMMC0_VSELE
E17   GND   NC   NC   NC
E19   GND   VDD_EMMC0_1P8_3   GND   VDD_EMMC0_1P8_3
E21   NC   VDD_ENET0_1P8_2   NC   NC
E23   GND   VDD_ESAI_SPDIF_   GND   VDD_ESAI_SPDIF_
E25   GND   VDD_ESAI_SPDIF_   GND   VDD_ESAI_SPDIF_
E27   GND   VDD_ESAI_SPDIF_   GND   VDD_ESAI_SPDIF_
E29   GND   VDD_SPI_MCLK_UA   GND   VDD_SPI_MCLK_UA
F2   GND   NC   NC   NC
F4   GND   NC   NC   NC
F6   GND   NC   NC   NC
F8   GND   NC   NC   NC
F10   NC   NC   NC   NC
F12   NC   NC   NC   NC
F14   GND   VDD_EMMC0_1P8_3   GND   VDD_EMMC0_1P8_3
F16   GND   VDD_EMMC0_VSELE   GND   VDD_EMMC0_VSELE
F18   GND   VDD_EMMC0_1P8_3   GND   VDD_EMMC0_1P8_3
F20   GND   VDD_ENET0_VSELE   GND   VDD_ENET0_VSELE
F22   GND   VDD_ENET_MDIO_1   GND   VDD_ENET_MDIO_1
F24   GND   VDD_ESAI_SPDIF_   GND   VDD_ESAI_SPDIF_
F26   NC   VDD_ENET_MDIO_1   NC   NC
F28   GND   VDD_SPI_MCLK_UA   GND   VDD_SPI_MCLK_UA
G1   GND   VDD_DDR_VDDQ   GND   VDD_DDR_VDDQ
G3   GND   VDD_DDR_VDDQ   GND   VDD_DDR_VDDQ
G5   GND   VDD_DDR_VDDQ   GND   VDD_DDR_VDDQ
G7   GND   VDD_DDR_VDDQ   GND   VDD_DDR_VDDQ
G9   GND   VDD_DDR_VDDQ   GND   VDD_DDR_VDDQ
G11   PCIE0_PHY_PLL_R NC   NC   NC
G13   GND   VDD_USB_3P3   GND   VDD_USB_3P3
G15   GND   VDD_EMMC0_1P8_3   GND   VDD_EMMC0_1P8_3
G17   GND   VDD_EMMC0_VSELE   GND   VDD_EMMC0_VSELE
G19   GND   VDD_ENET0_VSELE   GND   VDD_ENET0_VSELE
G21   GND   VDD_ENET0_1P8_2   GND   VDD_ENET0_1P8_2
G23   GND   VDD_ESAI_SPDIF_   GND   VDD_ESAI_SPDIF_
G25   GND   VDD_SPI_MCLK_UA   GND   VDD_SPI_MCLK_UA
G27   GND   VDD_SPI_MCLK_UA   GND   VDD_SPI_MCLK_UA
G29   GND   VDD_SPI_MCLK_UA   GND   VDD_SPI_MCLK_UA
H2   GND   VDD_DDR_VDDQ   GND   VDD_DDR_VDDQ
H4   GND   VDD_DDR_VDDQ   GND   VDD_DDR_VDDQ
H6   GND   VDD_DDR_VDDQ   GND   VDD_DDR_VDDQ
H8   GND   VDD_DDR_VDDQ   GND   VDD_DDR_VDDQ
H10   GND   VDD_DDR_VDDQ   GND   VDD_DDR_VDDQ
H12   NC   NC   NC   NC
H14   GND   VDD_USB_3P3   GND   VDD_USB_3P3
H16   GND   VDD_EMMC0_VSELE   GND   VDD_EMMC0_VSELE
H18   GND   VDD_ENET0_VSELE   GND   VDD_ENET0_VSELE
H20   GND   VDD_ENET0_1P8_2   GND   VDD_ENET0_1P8_2
H22   GND   VDD_ESAI_SPDIF_   GND   VDD_ESAI_SPDIF_
H24   GND   VDD_SPI_MCLK_UA   GND   VDD_SPI_MCLK_UA
H26   GND   NC   NC   NC
H28   GND   VDD_SPI_MCLK_UA   GND   VDD_SPI_MCLK_UA
J1   GND   NC   NC   NC
J3   GND   NC   NC   NC
J5   GND   NC   NC   NC
J7   GND   NC   NC   NC
J9   NC   VDD_PCIE_DIG_1P   NC   NC
J11   NC   VDD_PCIE_1P8   NC   NC
J13   GND   NC   NC   NC
J15   GND   VDD_USB_1P8   GND   VDD_USB_1P8
J17   GND   VDD_EMMC0_VSELE   GND   VDD_EMMC0_VSELE
J19   GND   VDD_ENET0_VSELE   GND   VDD_ENET0_VSELE
J21   GND   VDD_ENET_MDIO_1   GND   VDD_ENET_MDIO_1
J23   GND   VDD_ESAI_SPDIF_   GND   VDD_ESAI_SPDIF_
J25   GND   VDD_SPI_MCLK_UA   GND   VDD_SPI_MCLK_UA
J27   GND   VDD_SPI_MCLK_UA   GND   VDD_SPI_MCLK_UA
J29   GND   VDD_SPI_MCLK_UA   GND   VDD_SPI_MCLK_UA
K2   GND   VDD_DDR_VDDQ   GND   VDD_DDR_VDDQ
K4   GND   VDD_DDR_VDDQ   GND   VDD_DDR_VDDQ
K6   GND   VDD_DDR_VDDQ   GND   VDD_DDR_VDDQ
K8   NC   VDD_DDR_VDDQ   NC   NC
K10   NC   VDD_ANA0_1P8   NC   NC
K12   NC   VDD_PCIE_LDO_1P   NC   NC
K14   NC   VDD_USB_1P8   NC   NC
K16   NC   VDD_MAIN   NC   NC
K18   GND   NC   NC   NC
K20   NC   VDD_GPU   NC   NC
K22   GND   VDD_ESAI_SPDIF_   GND   VDD_ESAI_SPDIF_
K24   GND   VDD_SPI_MCLK_UA   GND   VDD_SPI_MCLK_UA
K26   NC   VDD_ESAI_SPDIF_   NC   NC
K28   GND   VDD_SPI_MCLK_UA   GND   VDD_SPI_MCLK_UA
L1   GND   VDD_DDR_VDDQ   GND   VDD_DDR_VDDQ
L3   GND   VDD_DDR_VDDQ   GND   VDD_DDR_VDDQ
L5   GND   VDD_DDR_VDDQ   GND   VDD_DDR_VDDQ
L7   GND   VDD_DDR_VDDQ   GND   VDD_DDR_VDDQ
L9   GND   NC   NC   NC
L11   GND   NC   NC   NC
L13   NC   VDD_MAIN   NC   NC
L15   GND   NC   NC   NC
L17   NC   VDD_GPU   NC   NC
L19   NC   VDD_GPU   NC   NC
L21   NC   VDD_MAIN   NC   NC
L23   GND   VDD_SPI_MCLK_UA   GND   VDD_SPI_MCLK_UA
L25   GND   VDD_SPI_MCLK_UA   GND   VDD_SPI_MCLK_UA
L27   NC   VDD_SPI_MCLK_UA   NC   NC
L29   GND   NC   NC   NC
M2   GND   NC   NC   NC
M4   GND   NC   NC   NC
M6   GND   NC   NC   NC
M8   NC   VDD_DDR_VDDQ   NC   NC
M10   NC   VDD_MAIN   NC   NC
M12   GND   NC   NC   NC
M14   NC   VDD_MAIN   NC   NC
M16   GND   NC   NC   NC
M18   NC   VDD_GPU   NC   NC
M20   GND   NC   NC   NC
M22   GND   VDD_SPI_MCLK_UA   GND   VDD_SPI_MCLK_UA
M24   GND   NC   NC   NC
M26   GND   NC   NC   NC
M28   NC   ADC_VREFH   NC   NC
N1   GND   VDD_DDR_VDDQ   GND   VDD_DDR_VDDQ
N3   GND   VDD_DDR_VDDQ   GND   VDD_DDR_VDDQ
N5   GND   VDD_DDR_VDDQ   GND   VDD_DDR_VDDQ
N7   GND   VDD_DDR_VDDQ   GND   VDD_DDR_VDDQ
N9   NC   VDD_DDR_VDDQ   NC   NC
N11   NC   VDD_MAIN   NC   NC
N13   GND   NC   NC   NC
N15   NC   VDD_MAIN   NC   NC
N17   GND   NC   NC   NC
N19   NC   VDD_GPU   NC   NC
N21   GND   NC   NC   NC
N23   GND   VDD_ADC_DIG_1P8   GND   VDD_ADC_DIG_1P8
N25   GND   VDD_ADC_DIG_1P8   GND   VDD_ADC_DIG_1P8
N27   GND   VDD_ADC_DIG_1P8   GND   VDD_ADC_DIG_1P8
N29   ADC_VREFL   NC   NC   NC
P2   GND   VDD_DDR_VDDQ   GND   VDD_DDR_VDDQ
P4   GND   VDD_DDR_VDDQ   GND   VDD_DDR_VDDQ
P6   GND   VDD_DDR_VDDQ   GND   VDD_DDR_VDDQ
P8   NC   VDD_DDR_VDDQ   NC   NC
P10   GND   NC   NC   NC
P12   NC   VDD_MAIN   NC   NC
P14   GND   NC   NC   NC
P16   NC   VDD_MAIN   NC   NC
P18   GND   NC   NC   NC
P20   NC   VDD_GPU   NC   NC
P22   NC   VDD_ADC_1P8   NC   NC
P24   GND   VDD_ADC_DIG_1P8   GND   VDD_ADC_DIG_1P8
P26   GND   VDD_ADC_DIG_1P8   GND   VDD_ADC_DIG_1P8
P28   GND   VDD_ADC_DIG_1P8   GND   VDD_ADC_DIG_1P8
R1   GND   NC   NC   NC
R3   GND   NC   NC   NC
R5   GND   NC   NC   NC
R7   GND   NC   NC   NC
R9   GND   NC   NC   NC
R11   GND   NC   NC   NC
R13   NC   VDD_MAIN   NC   NC
R15   GND   NC   NC   NC
R17   NC   VDD_GPU   NC   NC
R19   GND   NC   NC   NC
R21   NC   VDD_MAIN   NC   NC
R23   GND   NC   NC   NC
R25   GND   NC   NC   NC
R27   GND   NC   NC   NC
R29   GND   NC   NC   NC
T2   GND   VDD_DDR_VDDQ   GND   VDD_DDR_VDDQ
T4   GND   VDD_DDR_VDDQ   GND   VDD_DDR_VDDQ
T6   GND   VDD_DDR_VDDQ   GND   VDD_DDR_VDDQ
T8   NC   VDD_DDR_VDDQ   NC   NC
T10   NC   VDD_MAIN   NC   NC
T12   GND   NC   NC   NC
T14   NC   VDD_MAIN   NC   NC
T16   GND   NC   NC   NC
T18   NC   VDD_GPU   NC   NC
T20   GND   NC   NC   NC
T22   GND   VDD_CAN_UART_1P   GND   VDD_CAN_UART_1P
T24   GND   VDD_CAN_UART_1P   GND   VDD_CAN_UART_1P
T26   NC   VDD_ADC_DIG_1P8   NC   NC
T28   GND   VDD_CAN_UART_1P   GND   VDD_CAN_UART_1P
U1   GND   VDD_DDR_VDDQ   GND   VDD_DDR_VDDQ
U3   GND   VDD_DDR_VDDQ   GND   VDD_DDR_VDDQ
U5   GND   VDD_DDR_VDDQ   GND   VDD_DDR_VDDQ
U7   GND   VDD_DDR_VDDQ   GND   VDD_DDR_VDDQ
U9   NC   VDD_DDR_VDDQ   NC   NC
U11   NC   VDD_MAIN   NC   NC
U13   GND   NC   NC   NC
U15   NC   VDD_MAIN   NC   NC
U17   GND   NC   NC   NC
U19   NC   VDD_MAIN   NC   NC
U21   NC   VDD_CAN_UART_1P   NC   NC
U23   GND   VDD_CAN_UART_1P   GND   VDD_CAN_UART_1P
U25   GND   VDD_CAN_UART_1P   GND   VDD_CAN_UART_1P
U27   GND   VDD_CAN_UART_1P   GND   VDD_CAN_UART_1P
U29   GND   VDD_CAN_UART_1P   GND   VDD_CAN_UART_1P
V2   GND   NC   NC   NC
V4   GND   NC   NC   NC
V6   GND   NC   NC   NC
V8   NC   VDD_DDR_VDDQ   NC   NC
V10   GND   NC   NC   NC
V12   NC   VDD_A35   NC   NC
V14   NC   VDD_A35   NC   NC
V16   NC   VDD_A35   NC   NC
V18   GND   NC   NC   NC
V20   NC   VDD_MAIN   NC   NC
V22   GND   VDD_CAN_UART_1P   GND   VDD_CAN_UART_1P
V24   GND   NC   NC   NC
V26   GND   VDD_CAN_UART_1P   GND   VDD_CAN_UART_1P
V28   GND   VDD_CAN_UART_1P   GND   VDD_CAN_UART_1P
W1   GND   VDD_DDR_VDDQ   GND   VDD_DDR_VDDQ
W3   GND   VDD_DDR_VDDQ   GND   VDD_DDR_VDDQ
W5   NC   NC   NC   NC
W7   NC   VDD_DDR_PLL_1P8   NC   NC
W9   GND   NC   NC   NC
W11   GND   NC   NC   NC
W13   NC   VDD_A35   NC   NC
W15   NC   VDD_A35   NC   NC
W17   NC   VDD_A35   NC   NC
W19   GND   NC   NC   NC
W21   NC   VDD_ANA1_1P8   NC   NC
W23   GND   VDD_ANA1_1P8   GND   VDD_ANA1_1P8
W25   GND   VDD_CAN_UART_1P   GND   VDD_CAN_UART_1P
W27   GND   VDD_CAN_UART_1P   GND   VDD_CAN_UART_1P
W29   GND   VDD_CAN_UART_1P   GND   VDD_CAN_UART_1P
Y2   GND   VDD_DDR_VDDQ   GND   VDD_DDR_VDDQ
Y4   GND   VDD_DDR_VDDQ   GND   VDD_DDR_VDDQ
Y6   NC   DDR_VREF   NC   NC
Y8   NC   VDD_DDR_VDDQ   NC   NC
Y10   NC   VDD_MAIN   NC   NC
Y12   GND   NC   NC   NC
Y14   NC   VDD_MAIN   NC   NC
Y16   GND   NC   NC   NC
Y18   NC   VDD_MAIN   NC   NC
Y20   GND   NC   NC   NC
Y22   GND   VDD_ANA1_1P8   GND   VDD_ANA1_1P8
Y24   GND   VDD_ANA1_1P8   GND   VDD_ANA1_1P8
Y26   NC   VDD_SNVS_4P2   NC   NC
Y28   GND   VDD_CAN_UART_1P   GND   VDD_CAN_UART_1P
AA1   GND   NC   NC   NC
AA3   GND   NC   NC   NC
AA5   GND   NC   NC   NC
AA7   GND   NC   NC   NC
AA9   NC   VDD_DDR_VDDQ   NC   NC
AA11   NC   VDD_MAIN   NC   NC
AA13   NC   VDD_MIPI_1P8   NC   NC
AA15   NC   VDD_MIPI_1P0   NC   NC
AA17   GND   NC   NC   NC
AA19   NC   VDD_MAIN   NC   NC
AA21   NC   VDD_TMPR_CSI_1P   NC   NC
AA23   GND   VDD_ANA1_1P8   GND   VDD_ANA1_1P8
AA25   GND   VDD_ANA1_1P8   GND   VDD_ANA1_1P8
AA27   GND   NC   NC   NC
AA29   GND   VDD_ANA1_1P8   GND   VDD_ANA1_1P8
AB2   GND   VDD_DDR_VDDQ   GND   VDD_DDR_VDDQ
AB4   GND   VDD_DDR_VDDQ   GND   VDD_DDR_VDDQ
AB6   GND   VDD_DDR_VDDQ   GND   VDD_DDR_VDDQ
AB8   NC   VDD_DDR_VDDQ   NC   NC
AB10   GND   VDD_QSPI0A_1P8_   GND   VDD_QSPI0A_1P8_
AB12   GND   VDD_QSPI0A_1P8_   GND   VDD_QSPI0A_1P8_
AB14   NC   VDD_MIPI_1P8   NC   NC
AB16   NC   VDD_MIPI_1P0   NC   NC
AB18   NC   VDD_MIPI_CSI_DI   NC   NC
AB20   GND   VDD_SNVS_LDO_1P   GND   VDD_SNVS_LDO_1P
AB22   GND   VDD_ANA1_1P8   GND   VDD_ANA1_1P8
AB24   GND   VDD_ANA1_1P8   GND   VDD_ANA1_1P8
AB26   NC   VDD_SNVS_LDO_1P   NC   NC
AB28   GND   VDD_ANA1_1P8   GND   VDD_ANA1_1P8
AC1   GND   VDD_DDR_VDDQ   GND   VDD_DDR_VDDQ
AC3   GND   VDD_DDR_VDDQ   GND   VDD_DDR_VDDQ
AC5   GND   VDD_DDR_VDDQ   GND   VDD_DDR_VDDQ
AC7   GND   VDD_QSPI0B_1P8_   GND   VDD_QSPI0B_1P8_
AC9   GND   VDD_QSPI0A_1P8_   GND   VDD_QSPI0A_1P8_
AC11   GND   VDD_MIPI_1P8   GND   VDD_MIPI_1P8
AC13   GND   VDD_MIPI_1P8   GND   VDD_MIPI_1P8
AC15   GND   VDD_MIPI_1P8   GND   VDD_MIPI_1P8
AC17   GND   VDD_MIPI_1P8   GND   VDD_MIPI_1P8
AC19   GND   VDD_MIPI_1P8   GND   VDD_MIPI_1P8
AC21   GND   VDD_TMPR_CSI_1P   GND   VDD_TMPR_CSI_1P
AC23   GND   VDD_ANA1_1P8   GND   VDD_ANA1_1P8
AC25   GND   VDD_ANA1_1P8   GND   VDD_ANA1_1P8
AC27   GND   VDD_ANA1_1P8   GND   VDD_ANA1_1P8
AC29   GND   VDD_ANA1_1P8   GND   VDD_ANA1_1P8
AD2   GND   NC   NC   NC
AD4   GND   NC   NC   NC
AD6   GND   NC   NC   NC
AD8   NC   VDD_QSPI0A_1P8_   NC   NC
AD10   GND   VDD_QSPI0A_1P8_   GND   VDD_QSPI0A_1P8_
AD12   GND   VDD_MIPI_1P8   GND   VDD_MIPI_1P8
AD14   GND   VDD_MIPI_1P8   GND   VDD_MIPI_1P8
AD16   GND   VDD_MIPI_1P8   GND   VDD_MIPI_1P8
AD18   GND   VDD_MIPI_1P8   GND   VDD_MIPI_1P8
AD20   GND   VDD_MIPI_1P8   GND   VDD_MIPI_1P8
AD22   GND   VDD_TMPR_CSI_1P   GND   VDD_TMPR_CSI_1P
AD24   GND   NC   NC   NC
AD26   GND   VDD_ANA1_1P8   GND   VDD_ANA1_1P8
AD28   GND   VDD_ANA1_1P8   GND   VDD_ANA1_1P8
AE1   GND   VDD_QSPI0B_1P8_   GND   VDD_QSPI0B_1P8_
AE3   GND   VDD_QSPI0B_1P8_   GND   VDD_QSPI0B_1P8_
AE5   NC   VDD_QSPI0B_1P8_   NC   NC
AE7   GND   VDD_QSPI0B_1P8_   GND   VDD_QSPI0B_1P8_
AE9   GND   NC   NC   NC
AE11   GND   NC   NC   NC
AE13   GND   NC   NC   NC
AE15   GND   NC   NC   NC
AE17   GND   NC   NC   NC
AE19   GND   NC   NC   NC
AE21   GND   NC   NC   NC
AE23   NC   NC   NC   NC
AE25   GND   VDD_ANA1_1P8   GND   VDD_ANA1_1P8
AE27   GND   NC   NC   NC
AE29   GND   VDD_ANA1_1P8   GND   VDD_ANA1_1P8
AF2   GND   VDD_QSPI0B_1P8_   GND   VDD_QSPI0B_1P8_
AF4   GND   VDD_QSPI0B_1P8_   GND   VDD_QSPI0B_1P8_
AF6   GND   VDD_QSPI0B_1P8_   GND   VDD_QSPI0B_1P8_
AF8   GND   VDD_MIPI_1P8   GND   VDD_MIPI_1P8
AF10   GND   VDD_MIPI_1P8   GND   VDD_MIPI_1P8
AF12   GND   VDD_MIPI_1P8   GND   VDD_MIPI_1P8
AF14   GND   VDD_MIPI_1P8   GND   VDD_MIPI_1P8
AF16   GND   VDD_MIPI_1P8   GND   VDD_MIPI_1P8
AF18   GND   VDD_MIPI_CSI_DI   GND   VDD_MIPI_CSI_DI
AF20   GND   VDD_TMPR_CSI_1P   GND   VDD_TMPR_CSI_1P
AF22   NC   VDD_CSI_1P8_3P3   NC   NC
AF24   NC   NC   NC   NC
AF26   GND   VDD_SNVS_LDO_1P   GND   VDD_SNVS_LDO_1P
AF28   GND   VDD_ANA1_1P8   GND   VDD_ANA1_1P8
AG1   GND   NC   NC   NC
AG3   GND   VDD_QSPI0A_1P8_   GND   VDD_QSPI0A_1P8_
AG5   GND   VDD_QSPI0A_1P8_   GND   VDD_QSPI0A_1P8_
AG7   GND   VDD_MIPI_1P8   GND   VDD_MIPI_1P8
AG9   GND   VDD_MIPI_1P8   GND   VDD_MIPI_1P8
AG11   GND   VDD_MIPI_1P8   GND   VDD_MIPI_1P8
AG13   GND   VDD_MIPI_1P8   GND   VDD_MIPI_1P8
AG15   GND   VDD_MIPI_1P8   GND   VDD_MIPI_1P8
AG17   GND   NC   NC   NC
AG19   GND   VDD_CSI_1P8_3P3   GND   VDD_CSI_1P8_3P3
AG21   GND   VDD_TMPR_CSI_1P   GND   VDD_TMPR_CSI_1P
AG23   GND   VDD_TMPR_CSI_1P   GND   VDD_TMPR_CSI_1P
AG25   GND   NC   NC   NC
AG27   GND   NC   NC   NC
AG29   GND   NC   NC   NC
AH2   GND   VDD_QSPI0B_1P8_   GND   VDD_QSPI0B_1P8_
AH4   GND   VDD_QSPI0A_1P8_   GND   VDD_QSPI0A_1P8_
AH6   GND   NC   NC   NC
AH8   GND   VDD_MIPI_1P8   GND   VDD_MIPI_1P8
AH10   GND   VDD_MIPI_1P8   GND   VDD_MIPI_1P8
AH12   GND   VDD_MIPI_1P8   GND   VDD_MIPI_1P8
AH14   GND   VDD_MIPI_1P8   GND   VDD_MIPI_1P8
AH16   GND   VDD_MIPI_1P8   GND   VDD_MIPI_1P8
AH18   GND   VDD_CSI_1P8_3P3   GND   VDD_CSI_1P8_3P3
AH20   GND   VDD_TMPR_CSI_1P   GND   VDD_TMPR_CSI_1P
AH22   GND   VDD_TMPR_CSI_1P   GND   VDD_TMPR_CSI_1P
AH24   GND   VDD_TMPR_CSI_1P   GND   VDD_TMPR_CSI_1P
AH26   GND   VDD_SNVS_LDO_1P   GND   VDD_SNVS_LDO_1P
AH28   GND   VDD_ANA1_1P8   GND   VDD_ANA1_1P8
AJ3   GND   NC   NC   NC
AJ5   GND   VDD_QSPI0A_1P8_   GND   VDD_QSPI0A_1P8_
AJ7   GND   VDD_MIPI_1P8   GND   VDD_MIPI_1P8
AJ9   GND   VDD_MIPI_1P8   GND   VDD_MIPI_1P8
AJ11   GND   VDD_MIPI_1P8   GND   VDD_MIPI_1P8
AJ13   GND   VDD_MIPI_1P8   GND   VDD_MIPI_1P8
AJ15   GND   VDD_MIPI_1P8   GND   VDD_MIPI_1P8
AJ17   GND   VDD_CSI_1P8_3P3   GND   VDD_CSI_1P8_3P3
AJ19   GND   VDD_CSI_1P8_3P3   GND   VDD_CSI_1P8_3P3
AJ21   GND   VDD_TMPR_CSI_1P   GND   VDD_TMPR_CSI_1P
AJ23   GND   VDD_TMPR_CSI_1P   GND   VDD_TMPR_CSI_1P
AJ25   GND   VDD_SNVS_LDO_1P   GND   VDD_SNVS_LDO_1P
AJ27   GND   NC   NC   NC
[Diff Pin] inv_pin   vdiff   tdelay_typ   tdelay_min   tdelay_max
AE23   AF24   NA   NA   NA   NA
H2   G3   NA   NA   NA   NA
A7   B8   NA   NA   NA   NA
U3   U1   NA   NA   NA   NA
U5   T4   NA   NA   NA   NA
AD16   AC15   NA   NA   NA   NA
AD18   AC17   NA   NA   NA   NA
AD14   AC13   NA   NA   NA   NA
AD20   AC19   NA   NA   NA   NA
AD12   AC11   NA   NA   NA   NA
AH14   AF14   NA   NA   NA   NA
AJ15   AG15   NA   NA   NA   NA
AJ13   AG13   NA   NA   NA   NA
AH16   AF16   NA   NA   NA   NA
AH12   AF12   NA   NA   NA   NA
AJ9   AG9   NA   NA   NA   NA
AH8   AF8   NA   NA   NA   NA
AH10   AF10   NA   NA   NA   NA
AJ7   AG7   NA   NA   NA   NA
AJ11   AG11   NA   NA   NA   NA
A15   B16   NA   NA   NA   NA
A13   B12   NA   NA   NA   NA
D14   C13   NA   NA   NA   NA
A19   B18   NA   NA   NA   NA
|*   Model Selector   *
[Model Selector]  3V3SF_1V8_3V3_FCGPIO
BDPROGSCARUDQP_SDMMC_3V3SF_00   PSW=0 PDRV=0 MODE=1V8 SD & MMC
BDPROGSCARUDQP_SDMMC_3V3SF_01   PSW=0 PDRV=1 MODE=1V8 SD & MMC
BDPROGSCARUDQP_SDMMC_3V3SF_10   PSW=1 PDRV=0 MODE=3V3 SD & 3V3 MMC
BDPROGSCARUDQP_SDMMC_3V3SF_11   PSW=1 PDRV=1 MODE=3V3 SD & 3V3 MMC
BDPROGSCARUDQP_SDMMC_3V3SF_11_2v7   PSW=1 PDRV=1 MODE=2V7 SD & 2V7 MMC
BDPROGSCARUDQP_SDMMC_3V3SF_10_2v7   PSW=1 PDRV=0 MODE=2V7 SD & 2V7 MMC
[Model Selector] RGMIIRX_GPIO
RGMII_RX_2V5_mi   RGMII, 2.5V, RX-mode
BDPROGSCARUDQP_SDMMC_3V3SF_00   PSW=0 PDRV=0 MODE=1V8 SD & MMC
BDPROGSCARUDQP_SDMMC_3V3SF_01   PSW=0 PDRV=1 MODE=1V8 SD & MMC
BDPROGSCARUDQP_SDMMC_3V3SF_10   PSW=1 PDRV=0 MODE=3V3 SD & 3V3 MMC
BDPROGSCARUDQP_SDMMC_3V3SF_11   PSW=1 PDRV=1 MODE=3V3 SD & 3V3 MMC
BDPROGSCARUDQP_SDMMC_3V3SF_11_2v7   PSW=1 PDRV=1 MODE=2V7 SD & 2V7 MMC
BDPROGSCARUDQP_SDMMC_3V3SF_10_2v7   PSW=1 PDRV=0 MODE=2V7 SD & 2V7 MMC
[Model Selector] RGMIITX_GPIO
RGMII_TX_2V5_drv0_mo   RGMII, 2.5V, TX-mode, PDRV=low
RGMII_TX_2V5_drv1_mo   RGMII, 2.5V, TX-mode, PDRV=high
BDPROGSCARUDQP_SDMMC_3V3SF_00   PSW=0 PDRV=0 MODE=1V8 SD & MMC
BDPROGSCARUDQP_SDMMC_3V3SF_01   PSW=0 PDRV=1 MODE=1V8 SD & MMC
BDPROGSCARUDQP_SDMMC_3V3SF_10   PSW=1 PDRV=0 MODE=3V3 SD & 3V3 MMC
BDPROGSCARUDQP_SDMMC_3V3SF_11   PSW=1 PDRV=1 MODE=3V3 SD & 3V3 MMC
BDPROGSCARUDQP_SDMMC_3V3SF_11_2v7   PSW=1 PDRV=1 MODE=2V7 SD & 2V7 MMC
BDPROGSCARUDQP_SDMMC_3V3SF_10_2v7   PSW=1 PDRV=0 MODE=2V7 SD & 2V7 MMC
[Model Selector]  CSF_1V8_FCGPIO
BD_1mA   [DRIVE2=0  DRIVE1=0  DRIVE0=0  Drive Strength=1mA]
BD_2mA   [DRIVE2=0  DRIVE1=0  DRIVE0=1  Drive Strength=2mA]
BD_4mA   [DRIVE2=0  DRIVE1=1  DRIVE0=0  Drive Strength=4mA]
BD_6mA   [DRIVE2=0  DRIVE1=1  DRIVE0=1  Drive Strength=6mA]
BD_8mA   [DRIVE2=1  DRIVE1=0  DRIVE0=0  Drive Strength=8mA]
BD_10mA   [DRIVE2=1  DRIVE1=0  DRIVE0=1  Drive Strength=10mA]
BD_12mA   [DRIVE2=1  DRIVE1=1  DRIVE0=0  Drive Strength=12mA]
BD_HS   [DRIVE2=1  DRIVE1=1  DRIVE0=1  High Speed Cell]
[Model Selector] PCK_PAD
DWC_D5MCK3L_34   DDR3L DWC_D5M_PCK cell  Z0=34-Ohm
DWC_D5MCK3L_40   DDR3L DWC_D5M_PCK cell  Z0=40-Ohm
DWC_D5MCK3L_48   DDR3L DWC_D5M_PCK cell  Z0=48-Ohm
DWC_D5MCKL4_40   LPDDR4 DWC_D5M_PCK cell  Z0=40-Ohm Driver SR=00
DWC_D5MCKL4_48   LPDDR4 DWC_D5M_PCK cell  Z0=48-Ohm Driver SR=00
DWC_D5MCKL4_60   LPDDR4 DWC_D5M_PCK cell  Z0=60-Ohm Driver SR=00
DWC_D5MCKL4_80   LPDDR4 DWC_D5M_PCK cell  Z0=80-Ohm Driver SR=00
[Model Selector] PCKE_PAD
DWC_D5MC3L_34   DDR3L DWC_D5M_PCKE cell  Z0=34-Ohm
DWC_D5MC3L_40   DDR3L DWC_D5M_PCKE cell  Z0=40-Ohm
DWC_D5MC3L_48   DDR3L DWC_D5M_PCKE cell  Z0=48-Ohm
DWC_D5MCL4_40   LPDDR4 DWC_D5M_PCKE cell  Z0=40-Ohm Driver SR=00
DWC_D5MCL4_48   LPDDR4 DWC_D5M_PCKE cell  Z0=48-Ohm Driver SR=00
DWC_D5MCL4_60   LPDDR4 DWC_D5M_PCKE cell  Z0=60-Ohm Driver SR=00
DWC_D5MCL4_80   LPDDR4 DWC_D5M_PCKE cell  Z0=80-Ohm Driver SR=00
[Model Selector] PDDRIO_PAD
DWC_D5MP3L_34   DDR3L DWC_D5M_PDDRIO cell  Z0=34-Ohm
DWC_D5MP3L_40   DDR3L DWC_D5M_PDDRIO cell  Z0=40-Ohm
DWC_D5MP3L_48   DDR3L DWC_D5M_PDDRIO cell  Z0=48-Ohm
DWC_D5MP3L_ODT40   DDR3L DWC_D5M_PDDRIO cell 40-Ohm ODT Receiver
DWC_D5MP3L_ODT60   DDR3L DWC_D5M_PDDRIO cell 60-Ohm ODT Receiver
DWC_D5MP3L_ODTOFF   DDR3L DWC_D5M_PDDRIO cell ODT off Receiver
DWC_D5MPL4_40   LPDDR4 DWC_D5M_PDDRIO cell  Z0=40-Ohm Driver SR=00
DWC_D5MPL4_48   LPDDR4 DWC_D5M_PDDRIO cell  Z0=48-Ohm Driver SR=00
DWC_D5MPL4_60   LPDDR4 DWC_D5M_PDDRIO cell  Z0=60-Ohm Driver SR=00
DWC_D5MPL4_80   LPDDR4 DWC_D5M_PDDRIO cell  Z0=80-Ohm Driver SR=00
DWC_D5MPL4_ODT40   LPDDR4 DWC_D5M_PDDRIO cell 40-Ohm ODT Receiver
DWC_D5MPL4_ODT48   LPDDR4 DWC_D5M_PDDRIO cell 48-Ohm ODT Receiver
DWC_D5MPL4_ODT60   LPDDR4 DWC_D5M_PDDRIO cell 60-Ohm ODT Receiver
DWC_D5MPL4_ODT80   LPDDR4 DWC_D5M_PDDRIO cell 80-Ohm ODT Receiver
DWC_D5MPL4_ODTOFF   LPDDR4 DWC_D5M_PDDRIO cell  ODT off Receiver
[Model Selector] PDQS_PAD
DWC_D5MPD3L_34   DDR3L DWC_D5M_PDQS cell  Z0=34-Ohm
DWC_D5MPD3L_40   DDR3L DWC_D5M_PDQS cell  Z0=40-Ohm
DWC_D5MPD3L_48   DDR3L DWC_D5M_PDQS cell  Z0=48-Ohm
DWC_D5MPD3L_ODT40   DDR3L DWC_D5M_PDQS cell 40-Ohm ODT Receiver
DWC_D5MPD3L_ODT60   DDR3L DWC_D5M_PDQS cell 60-Ohm ODT Receiver
DWC_D5MPD3L_ODTOFF   DDR3L DWC_D5M_PDQS cell ODT off Receiver
DWC_D5MPDL4_40   LPDDR4 DWC_D5M_PDQS cell  Z0=40-Ohm Driver SR=00
DWC_D5MPDL4_48   LPDDR4 DWC_D5M_PDQS cell  Z0=48-Ohm Driver SR=00
DWC_D5MPDL4_60   LPDDR4 DWC_D5M_PDQS cell  Z0=60-Ohm Driver SR=00
DWC_D5MPDL4_80   LPDDR4 DWC_D5M_PDQS cell  Z0=80-Ohm Driver SR=00
DWC_D5MPDL4_ODT40   LPDDR4 DWC_D5M_PDQS cell 40-Ohm ODT Receiver
DWC_D5MPDL4_ODT48   LPDDR4 DWC_D5M_PDQS cell 48-Ohm ODT Receiver
DWC_D5MPDL4_ODT60   LPDDR4 DWC_D5M_PDQS cell 60-Ohm ODT Receiver
DWC_D5MPDL4_ODT80   LPDDR4 DWC_D5M_PDQS cell 80-Ohm ODT Receiver
DWC_D5MPDL4_ODTOFF   LPDDR4 DWC_D5M_PDQS cell  ODT off Receiver
[Model Selector] MIPI_CSI
MIPI_HS_CSI   High Speed MIPI_CSI driver
MIPI_LP_CSI   Low Power MIPI_CSI driver
[Model Selector] MIPI_LVDS_DSI
MIPI_HS_DSI   High Speed MIPI_DSI driver
MIPI_LP_DSI   Low Power MIPI_DSI driver
LVDS_TX   LVDS driver
[Model Selector] 3V3SF_3V3_FCGPIO
BDPROG_00   [DRIVE0=0 DRIVE1=0]
BDPROG_01   [DRIVE0=0 DRIVE1=1]
BDPROG_10   [DRIVE0=1 DRIVE1=0]
BDPROG_11   [DRIVE0=1 DRIVE1=1]
[Model Selector] ABI_SERDES
abi_out   ABI Serdes output
abi_in   ABI Serdes input
[Model Selector] USB_NXP
hs_input   USB HS input
hs_ls_input   HSUSB LS input
hs_vbus_input   USB HS VBUS input
hsfs_host_input   FS input in host mode
hsfs_device_dp_input   FS dm input in device mode
hsfs_device_dm_input   FS dp input in device mode
hs_driver   HSUSB HS Driver
hs_fs_driver   HSUSB FS Driver
hs_ls_driver   HSUSB LS Driver
[Model Selector] IO_20UM_RES_ANAF
IO_20UM_RES_ANAF_1v8_mt   IO_20UM_RES_ANAF_FC_LIN_NXP, 1.8V
IO_20UM_RES_ANAF_3v3_mt   IO_20UM_RES_ANAF_FC_LIN_NXP, 3.3V
[Model Selector] IO_20UM_RES_ANAF_1V8
IO_20UM_RES_ANAF_1v8_mt   IO_20UM_RES_ANAF_FC_LIN_NXP, 1.8V
[Model Selector] PCIEREFCLKIO_P
DRIVER_P  PCIE REFCLK100M Positive Driver
RECEIVER_P  PCIE REFCLK100M Positive Receiver No ODT
[Model Selector] PCIEREFCLKIO_N
DRIVER_N  PCIE REFCLK100M Negative Driver
RECEIVER_N  PCIE REFCLK100M Negative Receiver No ODT
| Models and submodels in the file (87): BDPROGSCARUDQP_SDMMC_3V3SF_00 (I/O), BDPROGSCARUDQP_SDMMC_3V3SF_01 (I/O), BDPROGSCARUDQP_SDMMC_3V3SF_10_2v7 (I/O), BDPROGSCARUDQP_SDMMC_3V3SF_10 (I/O), BDPROGSCARUDQP_SDMMC_3V3SF_11_2v7 (I/O), BDPROGSCARUDQP_SDMMC_3V3SF_11 (I/O), BD_1mA (I/O), BD_2mA (I/O), BD_4mA (I/O), BD_6mA (I/O), BD_8mA (I/O), BD_10mA (I/O), BD_12mA (I/O), BD_HS (I/O), DWC_D5MCK3L_34 (I/O), DWC_D5MCK3L_40 (I/O), DWC_D5MCK3L_48 (I/O), DWC_D5MCKL4_40 (I/O), DWC_D5MCKL4_48 (I/O), DWC_D5MCKL4_60 (I/O), DWC_D5MCKL4_80 (I/O), DWC_D5MC3L_34 (I/O), DWC_D5MC3L_40 (I/O), DWC_D5MC3L_48 (I/O), DWC_D5MCL4_40 (I/O), DWC_D5MCL4_48 (I/O), DWC_D5MCL4_60 (I/O), DWC_D5MCL4_80 (I/O), DWC_D5MP3L_34 (I/O), DWC_D5MP3L_40 (I/O), DWC_D5MP3L_48 (I/O), DWC_D5MP3L_ODT40 (Input), DWC_D5MP3L_ODT60 (Input), DWC_D5MP3L_ODTOFF (Input), DWC_D5MPL4_40 (I/O), DWC_D5MPL4_48 (I/O), DWC_D5MPL4_60 (I/O), DWC_D5MPL4_80 (I/O), DWC_D5MPL4_ODT40 (Input), DWC_D5MPL4_ODT48 (Input), DWC_D5MPL4_ODT60 (Input), DWC_D5MPL4_ODT80 (Input), DWC_D5MPL4_ODTOFF (Input), DWC_D5MPD3L_34 (I/O), DWC_D5MPD3L_40 (I/O), DWC_D5MPD3L_48 (I/O), DWC_D5MPD3L_ODT40 (Input), DWC_D5MPD3L_ODT60 (Input), DWC_D5MPD3L_ODTOFF (Input), DWC_D5MPDL4_40 (I/O), DWC_D5MPDL4_48 (I/O), DWC_D5MPDL4_60 (I/O), DWC_D5MPDL4_80 (I/O), DWC_D5MPDL4_ODT40 (Input), DWC_D5MPDL4_ODT48 (Input), DWC_D5MPDL4_ODT60 (Input), DWC_D5MPDL4_ODT80 (Input), DWC_D5MPDL4_ODTOFF (Input), MIPI_HS_CSI (Input), MIPI_LP_CSI (Input), LVDS_TX (3-state), MIPI_HS_DSI (Output), MIPI_LP_DSI (I/O), BDPROG_00 (I/O), BDPROG_01 (I/O), BDPROG_10 (I/O), BDPROG_11 (I/O), abi_in (Input), abi_out (Output), RGMII_RX_2V5_mi (Input), RGMII_TX_2V5_drv0_mo (3-state), RGMII_TX_2V5_drv1_mo (3-state), hs_input (Input), hs_ls_input (Input), hs_vbus_input (Input), hsfs_host_input (Input), hsfs_device_dp_input (Input), hsfs_device_dm_input (Input), hs_driver (Output), hs_fs_driver (Output)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
